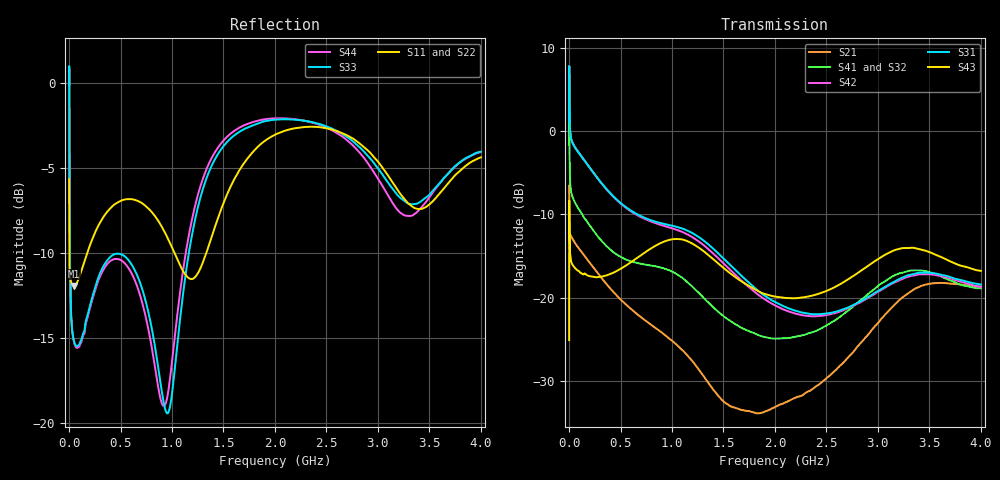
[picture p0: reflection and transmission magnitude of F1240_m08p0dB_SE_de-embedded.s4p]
! Integrated Device Technology
! Corporate Headquarters
! 6024 Silver Creek Valley Road
! San Jose, CA 95138  USA
! Phone:  1-408-284-8200
! Toll Free:  1-800-223-1366
! Webpage:  http://www.idt.com/
! Timing and RF Division
! 515 Groton Road, Suite 102
! Westford, MA 01886-6024
! Device:  F1240
! Description: Dual Intermediate Frequency Digital Variable Gain Amplifier
! Frequency:  10.0 -  500.00 MHz
! Package:  5x5 mm QFN Plastic Package: 32 pin
! Ports:  8 RF, 20 DC
!  Pin  1  = GA3 / Data  Pin 17  = RF OUT_B+
!  Pin  2  = GA4 / CLK  Pin 18  = RF OUT_B-
!  Pin  3  = GA5  Pin 19  = STBY_B
!  Pin  4  = VMODE  Pin 20  = Ground
!  Pin  5  = No Connect  Pin 21  = Ground
!  Pin  6  = GB5  Pin 22  = STB_A
!  Pin  7  = GB4  Pin 23  = RF OUT_A-  = Port 4
!  Pin  8  = GB3  Pin 24  = RF OUT_A+  = Port 3
!  Pin  9  = GB2  Pin 25  = GA0
!  Pin 10  = GB1  Pin 26  = ISET_A
!  Pin 11  = RF IN_B+  Pin 27  = VCC
!  Pin 12  = RF IN_B-  Pin 28  = Ground
!  Pin 13  = Ground  Pin 29  = RF IN_A-  = Port 2
!  Pin 14  = VCC  Pin 30  = RF IN_A+  = Port 1
!  Pin 15  = ISET_B  Pin 31  = GA1
!  Pin 16  = GB0  Pin 32  = GA2 / CSb
! Gain  = +19.5 dB
! State  = 1
! Voltage  = +5.00 V
! Current  = 85.292 mA (one channel only)
! Temperture  =  +25 C
! Test Date  =  2017-10-18
! Board  =  EB4031
! Data:  The device was measured on a custom evaluation board which has
!  individual transmission lines to the RF pins.  Data was collected
!  using a calibrated network analyzer.  The evaluation board was
!  de-embedded using Automatic Fixture Removal.
!  The reference plane is the edge of the package pin.
!  Only Channel A was measured.
!  This data is in single-ended operation.  If your needs are balanced
!  or differential S-parameters then this file needs to be used a
!  linear simulator.
! File Date:  2017-11-10  MJV
! Note:
!  Integrated Device Technology supplies this data as a sample of measured
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# Hz S dB R 100
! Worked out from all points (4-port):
!   410 points, 500 kHz to 4 GHz, reference 100 ohm
!   strongest paths, dB at 500 kHz, 930 MHz, 1.96 GHz, 2.98 GHz, 4 GHz:
!     S43: -25.1, -13.2, -19.8, -15.6, -16.8
!     S31: 1.1, -11.2, -20.3, -19.4, -18.4
!     S42: 1.1, -11.4, -20.7, -19.5, -18.8
!     S41: -1.6, -16.5, -24.9, -18.8, -18.9
!     S32: -1.6, -16.8, -24.7, -19.1, -19.2
!     S21: -6.5, -24.5, -33.4, -23.3, -18.7
!   lowest |S11| = -12.0 dB at 50 MHz (marker M1), VSWR 1.68, Z = 141 - j46.4 ohm
!   |S11| at or under -10 dB: 2.927 MHz to 177.6 MHz (174.6 MHz wide, 194 % of centre); 1.022 GHz to 1.334 GHz (311.7 MHz wide, 26.5 % of centre)
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500000  -5.68 -5.6  -6.54 -5.8  -31.57 77.8  -34.41 76.7
        -6.55 -5.8  -5.68 -5.6  -34.38 75.6  -31.56 78.9
        1.11 -110.7  -1.58 -112.6  -0.13 0.0  -25.12 -38.3
        -1.60 -111.5  1.10 -109.6  -25.12 -38.3  -0.14 2.3
3500000  -10.49 -22.2  -11.64 -20.0  -24.28 5.7  -29.50 -11.5
         -11.64 -20.0  -10.49 -22.3  -29.47 -11.7  -24.27 5.9
         4.09 157.0  -0.76 141.3  -4.01 -80.9  -10.34 178.7
         -0.79 141.5  4.09 157.2  -10.35 178.6  -4.06 -80.9
5e7  -11.96 -37.5  -13.30 -22.9  -25.61 -17.3  -32.68 -20.3
     -13.30 -22.9  -11.92 -38.1  -32.68 -20.3  -25.58 -17.4
     -1.81 151.9  -8.41 143.0  -15.25 -161.0  -16.38 153.4
     -8.40 143.1  -1.76 151.7  -16.35 153.3  -15.33 -161.6
5e8  -6.96 -144.2  -20.22 -124.5  -29.25 -101.4  -37.00 -90.8
     -20.23 -124.3  -6.91 -145.1  -37.12 -88.5  -29.54 -101.3
     -8.62 29.3  -15.21 -16.1  -10.08 -172.0  -16.63 16.0
     -15.11 -17.3  -8.70 27.8  -16.56 15.8  -10.43 -172.7
2.06e9  -2.91 -179.7  -32.70 60.9  -33.07 -22.5  -35.22 -0.6
        -32.83 61.4  -2.81 179.8  -35.82 5.9  -34.56 -16.4
        -20.91 60.8  -24.84 -6.6  -2.15 175.0  -20.22 32.5
        -24.91 -13.8  -21.31 63.6  -20.00 33.7  -2.09 171.9
2.92e9  -4.09 100.4  -24.22 -28.1  -28.64 -156.7  -30.92 -142.6
        -24.24 -28.2  -3.88 101.2  -31.48 -129.3  -30.05 -148.7
        -19.84 -71.5  -19.70 -151.7  -4.42 92.4  -16.83 -94.0
        -19.41 -163.4  -19.92 -68.1  -16.05 -91.8  -4.89 84.9
4e9  -4.39 -127.3  -18.68 120.6  -27.32 -24.8  -28.32 -9.7
     -18.68 120.6  -4.14 -126.0  -28.93 4.0  -29.16 -14.6
     -18.44 53.9  -19.19 -41.6  -4.06 -133.1  -18.22 61.9
     -18.89 -55.9  -18.75 60.1  -16.79 55.6  -4.07 -143.1
